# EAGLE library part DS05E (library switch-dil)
DIL/CODE SWITCH
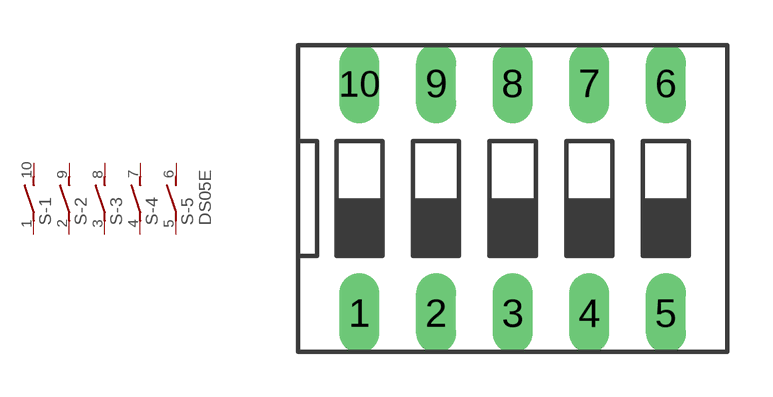
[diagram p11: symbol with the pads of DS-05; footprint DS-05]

Designator prefix S; gates -1=S -2=S -3=S -4=S -5=S+V

## DS05E (OC_FARNELL: unknown; OC_NEWARK: unknown)  [DS-05]
1  -1:1  pas
2  -2:1  pas
3  -3:1  pas
4  -4:1  pas
5  -5:1  pas
6  -5:2  pas
7  -4:2  pas
8  -3:2  pas
9  -2:2  pas
10  -1:2  pas

## Footprint DS-05 (pad centres in mm)
DIL/CODE SWITCH Mors distributor Buerklin, 17G556
drill 0.813 long: 1 -5.08,-3.81; 2 -2.54,-3.81; 3 0,-3.81; 4 2.54,-3.81; 5 5.08,-3.81; 6 5.08,3.81; 7 2.54,3.81; 8 0,3.81; 9 -2.54,3.81; 10 -5.08,3.81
